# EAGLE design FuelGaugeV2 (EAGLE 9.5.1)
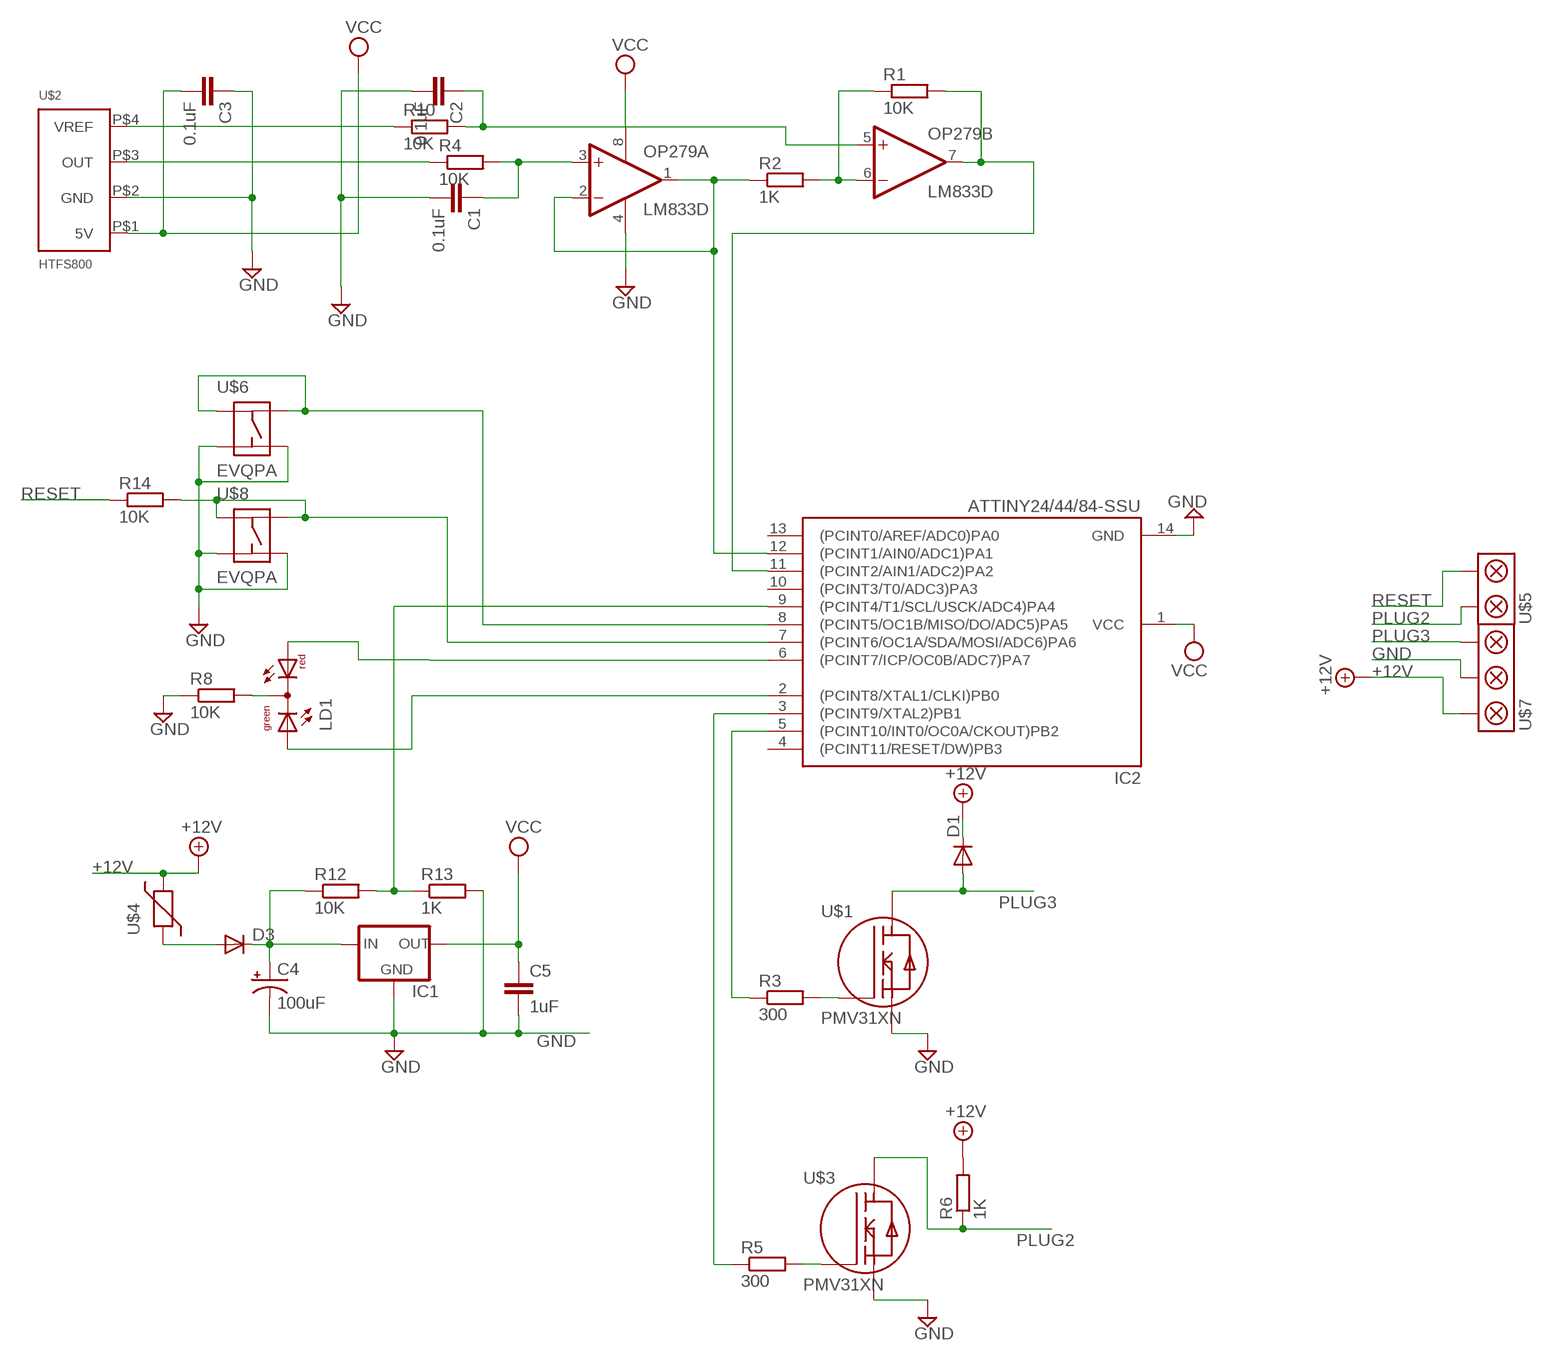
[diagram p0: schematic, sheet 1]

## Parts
C1  0.1uF  C-EUC1206  [C1206]
C2  0.1uF  C-EUC1206  [C1206]
C3  0.1uF  C-EUC1206  [C1206]
C4  100uF  CPOL-USD  [PANASONIC_D]
C5  1uF  C-EUC1206  [C1206]
D1  DIODE-SOD123  [SOD123]
D3  DIODE-SOD123  [SOD123]
IC1  78LXXSOT89  [SOT89R]
IC2  ATTINY24/44/84-SSU  [SOIC14]
LD1  DUOLED-RG-C  [DUOLED-C-5MM]
OP279  LM833D  [SO08]
R1  10K  R-EU_R1206  [R1206]
R2  1K  R-EU_R1206  [R1206]
R3  300  R-EU_R1206  [R1206]
R4  10K  R-EU_R1206  [R1206]
R5  300  R-EU_R1206  [R1206]
R6  1K  R-EU_R1206  [R1206]
R8  10K  R-EU_R1206  [R1206]
R10  10K  R-EU_R1206  [R1206]
R12  10K  R-EU_R1206  [R1206]
R13  1K  R-EU_R1206  [R1206]
R14  10K  R-EU_R1206  [R1206]
U$1  PMV31XN  [SOT23]
U$2  HTFS800  [HTFS800]
U$3  PMV31XN  [SOT23]
U$4  1206_POLYSWITCH  [1206]
U$5  SCREWTERM_2WAY  [SCREWTERM_3-5MM_2WAY]
U$6  EVQPA  [EVQPA]
U$7  SCREWTERM_3WAY  [SCREWTERM_3-5MM_3WAY]
U$8  EVQPA  [EVQPA]

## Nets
+12V: D1.C R6.2 U$4.P$2 U$7.P$3
ASDF: C4.+ D3.C IC1.1(IN) R12.1
GND: C1.2 C2.2 C3.1 C4.- C5.2 IC1.4(GND) IC2.14(GND) OP279.4(P:V-) R8.1 R13.2 U$1.P$2(S) U$2.P$2(GND) U$3.P$2(S) U$6.A U$6.A2 U$7.P$2 U$8.A U$8.A2
N$1: IC2.8((PCINT5/OC1B/MISO/DO/ADC5)PA5) U$6.B U$6.B2
N$2: IC2.12((PCINT1/AIN0/ADC1)PA1) OP279.1(A:OUT) OP279.2(A:-IN) R2.1
N$4: R3.2 U$1.P$1(G)
N$5: LD1.C R8.2
N$6: R4.1 U$2.P$3(OUT)
N$7: C1.1 OP279.3(A:+IN) R4.2
N$8: IC2.6((PCINT7/ICP/OC0B/ADC7)PA7) LD1.AR
N$9: IC2.9((PCINT4/T1/SCL/USCK/ADC4)PA4) R12.2 R13.1
N$10: OP279.6(B:-IN) R1.1 R2.2
N$11: IC2.2((PCINT8/XTAL1/CLKI)PB0) LD1.AX(AG)
N$12: IC2.11((PCINT2/AIN1/ADC2)PA2) OP279.7(B:OUT) R1.2
N$14: IC2.7((PCINT6/OC1A/SDA/MOSI/ADC6)PA6) R14.2 U$8.B U$8.B2
N$15: D3.A U$4.P$1
N$16: R5.2 U$3.P$1(G)
N$17: R10.1 U$2.P$4(VREF)
N$18: IC2.5((PCINT10/INT0/OC0A/CKOUT)PB2) R3.1
N$19: IC2.3((PCINT9/XTAL2)PB1) R5.1
N$23: C2.1 OP279.5(B:+IN) R10.2
PLUG2: R6.1 U$3.P$3(D) U$5.P$2
PLUG3: D1.A U$1.P$3(D) U$7.P$1
RESET: R14.1 U$5.P$1
VCC: C3.2 C5.1 IC1.2(OUT) IC2.1(VCC) OP279.8(P:V+) U$2.P$1(5V)
Unconnected: IC2.4((PCINT11/RESET/DW)PB3) IC2.10((PCINT3/T0/ADC3)PA3) IC2.13((PCINT0/AREF/ADC0)PA0)

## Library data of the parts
C1-C3 C5 = rcl:C-EU: CAPACITOR, European symbol
C4 = resistor:CPOL-US: POLARIZED CAPACITOR, American symbol
D1 D3 = diode:DIODE-: DIODE
IC1 = v-reg:78LXX: VOLTAGE REGULATOR
IC2 = ATtiny24-44-84:ATTINY24/44/84
LD1 = led:DUOLED-RG-C: DUO LED 2 colors (red/green), 5 mm, round, common Cathode www.ligitek.com or other producers.
OP279 = linear:LM833: OP AMP
R1-R6 R8 R10 R12-R14 = rcl:R-EU_: RESISTOR, European symbol
U$1 U$3 = Ians parts:PMV31XN
U$2 = Ians parts:HTFS800
U$4 = Ians parts:1206_POLYSWITCH
U$5 = Ians parts:SCREWTERM_2WAY
U$6 U$8 = Ians parts:EVQPA
U$7 = Ians parts:SCREWTERM_3WAY

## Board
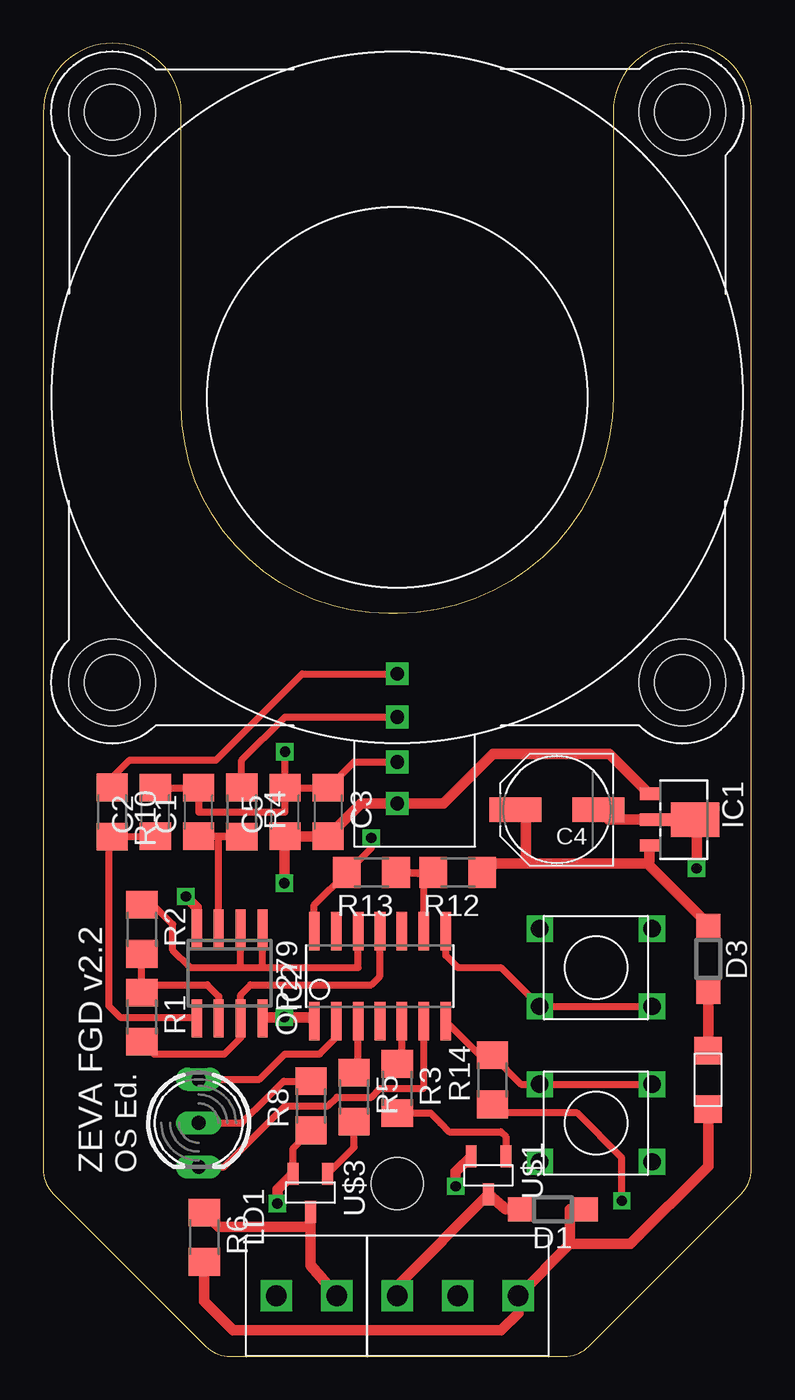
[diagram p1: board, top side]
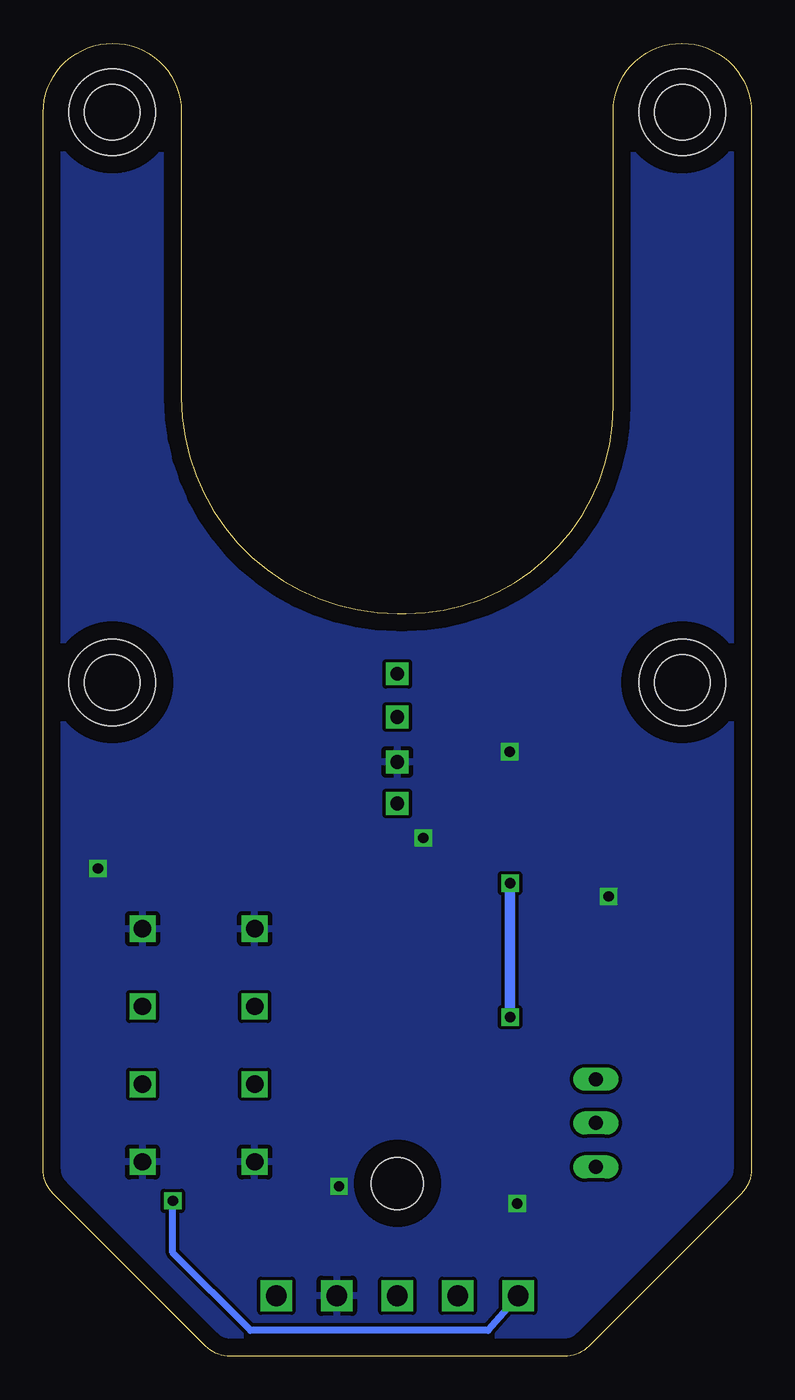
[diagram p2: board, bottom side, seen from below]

Size 41 x 76 mm. Coordinates in mm from the lower left corner, seen from the top.
Outline: 4.03,76 arc90 0,71.97 0,10.83 arc45 0.59,9.41 9.41,0.59 arc45 10.83,0 30.17,0 arc45 31.59,0.59 40.41,9.41 arc45 41,10.83 41,71.97 arc90 36.97,76 arc90 33,72.03 33,56 33,55.5 arc-90 20.5,43 20,43 arc-90 8,55 8,72.03 arc90 4.03,76
Copper layers (1*16): Top 0.035mm / dielectric 1.5mm / Bottom 0.035mm
Design rules "default *": minimum track width 10mil, minimum drill 10mil, track to track 8mil, track to pad 8mil, pad to pad 8mil, via to via 8mil, smd to smd 8mil, copper to edge 40mil, drill to drill 8mil, minimum pad ring 10mil, minimum via ring 8mil, stop-mask expansion 4mil, vias tented up to drill 0mil, thermal gap 10mil
Holes 5 mm at 4,39 37,39 4,72 37,72
Holes 3 mm at 20.5,10

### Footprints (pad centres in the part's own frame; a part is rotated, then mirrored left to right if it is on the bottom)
C1206 = smd 1.6 x 1.8: 1 -1.4,0; 2 1.4,0
PANASONIC_D = smd 3 x 1.4: + 2.4,0; - -2.4,0
SOD123 = smd 1.4 x 1.4: A 1.9,0; C -1.9,0
SOT89R = smd 0.7 x 1.1: 1 1.5,-1.75; 2 -1.5,-1.75 | smd 0.7 x 1.8: 3 0,-1.4 | smd 2 x 2.8: 4 0,0.9
SOIC14 = smd 0.61 x 2.21: 1 -3.81,-2.603; 2 -2.54,-2.603; 3 -1.27,-2.603; 4 0,-2.603; 5 1.27,-2.603; 6 2.54,-2.603; 7 3.81,-2.603; 8 3.81,2.603; 9 2.54,2.603; 10 1.27,2.603; 11 0,2.603; 12 -1.27,2.603; 13 -2.54,2.603; 14 -3.81,2.603
DUOLED-C-5MM = drill 0.813 long: AR 2.54,0; AX -2.54,0; C 0,0
SO08 = smd 0.6 x 2.2: 1 -1.905,-2.6; 2 -0.635,-2.6; 3 0.635,-2.6; 4 1.905,-2.6; 5 1.905,2.6; 6 0.635,2.6; 7 -0.635,2.6; 8 -1.905,2.6
R1206 = smd 1.6 x 1.803: 1 -1.422,0; 2 1.422,0
SOT23 = smd 1.27 x 0.635: P$1 -1.1,1; P$2 -1.1,-1; P$3 1.1,0
HTFS800 = drill 0.8 square: P$1 0,-23.5; P$2 0,-21.1; P$3 0,-18.5; P$4 0,-16 | hole 3.2: -16.5,16.5; 16.5,16.5; 16.5,-16.5; -16.5,-16.5
1206 = smd 1.6 x 1.6: P$1 -1.7,0; P$2 1.7,0
SCREWTERM_3-5MM_2WAY = drill 1.2 square: P$1 0,1.75; P$2 0,-1.75
EVQPA = drill 1 square: A -2.25,3.25; A2 -2.25,-3.25; B 2.25,3.25; B2 2.25,-3.25
SCREWTERM_3-5MM_3WAY = drill 1.2 square: P$1 0,3.5; P$2 0,0; P$3 0,-3.5

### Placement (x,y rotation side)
C1  9,31.5 90 top
C2  6.5,31.5 90 top
C3  16.5,31.5 270 top
C4  29.73,31.64 180 top
C5  14,31.5 90 top
D1  29.5,8.5 180 top
D3  38.5,23 270 top
IC1  36.83,31.06 270 top
IC2  19.5,22 0 top
LD1  9,13.5 270 top
OP279  10.79,22.17 180 top
R1  5.71,19.63 270 top
R2  5.71,24.71 270 top
R3  20.5,15.5 270 top
R4  11.5,31.5 270 top
R5  18,15 270 top
R6  9.33,6.89 270 top
R8  15.5,14.5 90 top
R10  4,31.5 270 top
R12  24,28 180 top
R13  19,28 180 top
R14  26,16 90 top
U$1  25.78,10.47 270 top
U$2  20.5,55.5 0 top
U$3  15.47,9.47 270 top
U$4  38.5,16 270 top
U$5  15.25,3.5 90 top
U$6  32,22.5 270 top
U$7  24,3.5 90 top
U$8  32,13.5 90 top

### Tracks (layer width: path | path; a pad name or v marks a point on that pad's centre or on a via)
+12V
  Top 0.61: U$4.P$2 38.5,11 34,6.5 30.5,6.5 | 30.5,6.5 U$7.P$3 27.5,2.5 26.5,1.5 11,1.5 9.33,3.17 R6.2 | D1.C 30.5,8.5 30.5,6.5
ASDF
  Top 0.61: 27.94,28.52 34.92,28.52 34.95,28.55 | IC1.1 35.08,28.68 34.95,28.55 | C4.+ 27.94,31.03 27.94,28.52 | 27.94,28.52 26.19,28.52 R12.1 | D3.C 38.5,25 34.95,28.55
GND  (via drill 0.6)
  Top 0.406: C5.2 v14,35 | C5.2 14,31.5 9,31.5 C1.2 C2.2 | v19,30 19,29.42 R13.2 15.69,26.11 IC2.14 | U$2.P$2 18,34.4 C3.1 C5.2 | R8.1 14.47,12.05 U$3.P$2
  Top 0.61: OP279.4 8.89,25.98 v8.26,26.61 | R13.2 17.78,27.89 | C4.- 32.71,31.06 IC1.4 37.83,30.96 v37.83,28.23 | v13.56,8.84 13.56,9.66 U$3.P$2 | v23.88,9.84 23.88,10.66 U$1.P$2
  pour Bottom: -1.27,-1.04 42.55,-1.04 42.55,76.86 -1.27,76.86
N$1
  Top 0.406: IC2.8 23.31,23.19 24,22.5 26.5,22.5 U$6.B2 U$6.B
N$2
  Top 0.406: R2.1 6.37,26.13 7.5,25 7.5,23.5 8.5,22.5 11.43,22.5 | 11.43,22.5 OP279.2 | 12.7,22.5 18.23,22.5 IC2.12 | 11.43,22.5 12.7,22.5 | 12.7,22.5 OP279.1
N$4
  Top 0.406: U$1.P$1 26.78,12.72 26.5,13 23.5,13 23,13.5 22.42,14.08 R3.2
N$5
  Top 0.406: LD1.C 11.5,13.5 13,15 13.92,15.92 R8.2
N$6
  Top 0.406: U$2.P$3 14,37 11.5,34.5 R4.1
N$7
  Top 0.406: C1.1 11.48,30.1 R4.2 10.16,30.08 OP279.3
N$8
  Top 0.406: LD1.AR 10.46,10.96 11,11.5 14,14.5 16.5,14.5 17,15 19,15 19.5,15.5 22,15.5 22.04,15.54 IC2.6
N$9
  Top 0.406: R12.2 R13.1 22.04,27.89 IC2.9
N$10
  Top 0.406: R2.2 R1.1 6.16,21.5 9.5,21.5 10.16,20.84 OP279.6
N$11
  Top 0.406: IC2.2 16.96,18.46 16,17.5 14,17.5 13,16.5 12.54,16.04 LD1.AX
N$12
  Top 0.406: IC2.11 19.5,22 19,21.5 12,21.5 11.43,20.93 OP279.7 11.43,18.43 10.5,17.5 6.42,17.5 R1.2
N$14
  Top 0.406: U$8.B2 U$8.B 27.67,15.75 R14.2 25.29,17.42 IC2.7
N$15
  Top 0.61: U$4.P$1 D3.A
N$16
  Top 0.406: U$3.P$1 18,12.1 R5.2
  Top 0.61: U$3.P$1 16.47,10.47
N$17
  Top 0.406: U$2.P$4 15,39.5 10,34.5 5,34.5 4,33.5 R10.1
N$18
  Top 0.406: IC2.5 20.77,16.62 R3.1
N$19
  Top 0.406: IC2.3 18.23,16.62 R5.1
N$23
  Top 0.406: OP279.5 8.83,19.63 4.45,19.63 3.81,20.27 3.81,30.08 R10.2 6.5,30.08 C2.1
PLUG2
  Top 0.61: 15.47,7.5 15.47,5.28 U$5.P$2 | 15.47,7.5 U$3.P$3 | R6.1 10.15,7.5 15.47,7.5
PLUG3
  Top 0.61: D1.A 26.78,8.5 U$1.P$3 20.5,4.09 U$7.P$1
RESET  (via drill 0.6)
  Top 0.406: v33.5,9 33.5,11.5 30.92,14.08 26.5,14.08 R14.1
  Bottom 0.406: U$5.P$1 15.25,1.5 29,1.5 33.5,6 v33.5,9
VCC  (via drill 0.6)
  Top 0.61: OP279.8 12.76,19.63 v13.97,19.63 15.46,19.63 IC2.1 | IC1.2 32.77,34.87 26.04,34.87 23.16,32 U$2.P$1 18.4,32 C3.2 C5.1 13.97,30.07 v13.97,27.39
  Bottom 0.61: v13.97,19.63 v13.97,27.39

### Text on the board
tPlace: ZEVA FGD v2.2 | OS Ed.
